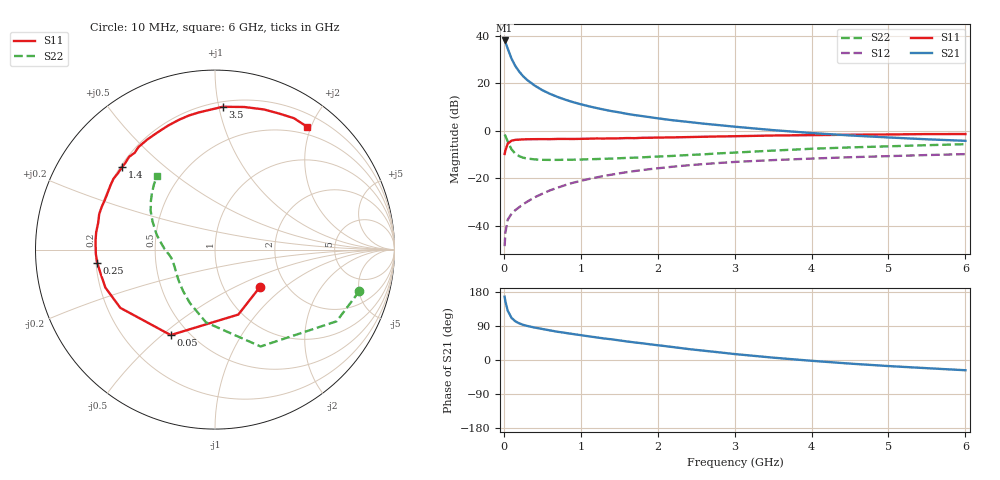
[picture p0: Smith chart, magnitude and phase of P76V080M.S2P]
! SIEMENS Small Signal Semiconductors
! BFP196
! Si NPN RF Bipolar Junction Transistor in SOT143
! VCE = 6 V  IC = 80 mA
! Common Emitter S-Parameters:  May  1996
# GHz  S  MA  R  50
!  f  S11  S21  S12  S22
! GHz  MAG  ANG  MAG  ANG  MAG  ANG  MAG  ANG
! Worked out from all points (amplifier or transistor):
!   36 points, 10 MHz to 6 GHz, reference 50 ohm
!   highest |S21| = 38.1 dB at 10 MHz (marker M1)
!   |S21| within 3 dB of that: start of sweep to 45.6 MHz
!   unconditionally stable (mu >= 1): 409.7 MHz to 4.658 GHz
!   at 250 MHz: K = 0.88, MSG = 27.0 dB, |S12| = -31.0 dB
!   at 1.4 GHz: K = 1.09, MAG = 11.6 dB, |S12| = -18.5 dB
!   at 6 GHz: K = 0.97, MSG = 2.8 dB, |S12| = -9.8 dB
!   S11 on the Smith chart (normalised r, x): 10 MHz: 1.47, -0.69; 50 MHz: 0.40, -0.53; 250 MHz: 0.21, -0.05; 1.4 GHz: 0.21, +0.37; 3.5 GHz: 0.24, +1.03; 6 GHz: 0.38, +1.94
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0.01  0.3256 -40.1  80.44 167.0  0.0037 77.6  0.8374 -16.0
0.02  0.3845 -70.2  74.14 154.6  0.0071 70.1  0.7867 -30.5
0.05  0.5364 -117.4  54.43 130.3  0.0133 54.2  0.5967 -64.8
0.1  0.6194 -148.4  33.19 111.1  0.0179 49.3  0.4083 -97.1
0.15  0.6464 -160.9  23.18 102.1  0.0213 51.0  0.3289 -115.2
0.2  0.6519 -168.6  17.73 96.7  0.0246 54.5  0.2925 -127.2
0.25  0.6602 -173.7  14.21 92.9  0.0283 56.7  0.2716 -136.3
0.3  0.6643 -177.9  11.92 90.1  0.0318 59.5  0.2616 -142.1
0.4  0.6676 175.7  9.019 85.6  0.0397 62.2  0.2497 -150.8
0.5  0.669 171.7  7.211 81.9  0.0471 63.8  0.2449 -156.5
0.6  0.6677 167.1  6.018 78.1  0.0556 64.2  0.2438 -160.4
0.7  0.6748 163.0  5.172 74.5  0.0634 64.0  0.2441 -163.4
0.9  0.6733 155.5  4.023 68.5  0.0805 62.6  0.2463 -167.7
1.1  0.6831 148.6  3.31 62.6  0.0961 60.8  0.2514 -170.8
1.4  0.6925 138.4  2.605 54.6  0.1191 57.0  0.2601 -174.7
1.7  0.701 129.6  2.15 46.3  0.1419 52.8  0.272 -178.8
2.2  0.7274 116.0  1.668 34.1  0.1754 45.2  0.296 174.7
2.8  0.7611 101.0  1.317 20.2  0.2102 36.2  0.3352 165.6
3.5  0.7969 86.9  1.035 6.2  0.2416 26.1  0.383 155.5
4.5  0.827 70.8  0.799 -9.5  0.2776 14.1  0.447 143.1
5.5  0.854 59.0  0.663 -21.6  0.3085 3.4  0.4983 133.0
6  0.8555 53.1  0.616 -27.0  0.3229 -2.2  0.5222 128.1
